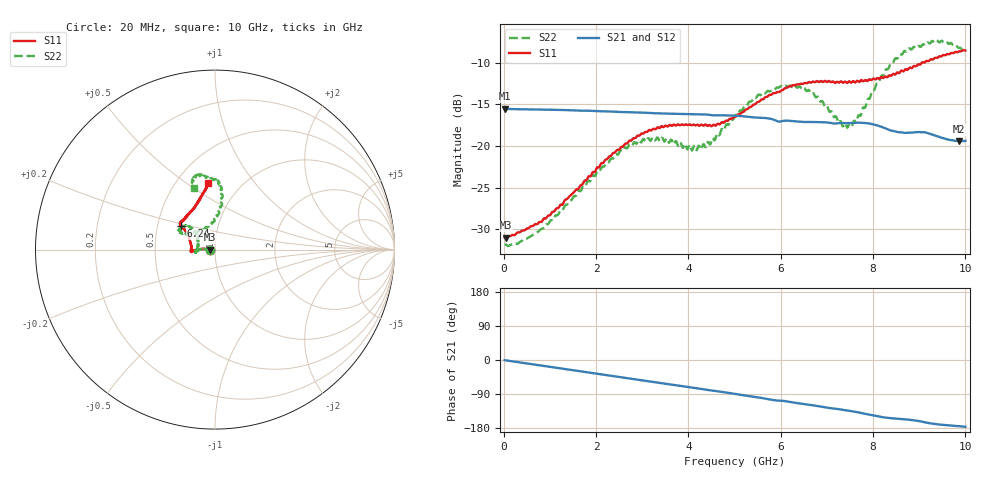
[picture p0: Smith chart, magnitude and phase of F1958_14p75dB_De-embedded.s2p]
! Integrated Device Technology
! Corporate Headquarters
! 6024 Silver Creek Valley Road
! San Jose, CA 95138  USA
! Phone:  1-408-284-8200
! Toll Free:  1-800-223-1366
! Webpage:  http://www.idt.com/
! Timing and RF Division
! 515 Groton Road, Suite 102
! Westford, MA 01886-6024
! Device:  F1958
! Description: 7-bit 0.25 dB Digital Step Attenuator
! Frequency:  0.001 -  6.000 GHz
! Package:  4x4 mm Thin QFN Plastic Package: 24 pin
! Ports:  2 RF, 12 DC
!  Pin  1  = D0
!  Pin  2  = VDD
!  Pin  3  = VMODE
!  Pin  4  = GND
!  Pin  5  = RF1  =  Port 1
!  Pin  6  = GND
!  Pin  7  = GND
!  Pin  8  = GND
!  Pin  9  = GND
!  Pin 10  = GND
!  Pin 11  = GND
!  Pin 12  = GND
!  Pin 13  = GND
!  Pin 14  = RF2  =  Port 2
!  Pin 15  = GND
!  Pin 16  = LE
!  Pin 17  = CLK
!  Pin 18  = DATA
!  Pin 19  = D6
!  Pin 20  = D5
!  Pin 21  = D4
!  Pin 22  = D3
!  Pin 23  = D2
!  Pin 24  = D1
! State:  59
! Atten State:  14.75 dB
! Voltage:  +3.30 Volts
! Current:  0.258 mA
! Data:  The device was measured on a F1958 evaluation board which has
!  individual transmission lines to the RF pins.  Data was collected
!  using a calibrated network analyzer.  The evaluation board was
!  de-embedded using Automatic Fixture Removal (AFR).
!  The reference plane is the edge of the package pin.
! Misc:
!  Action Tracker AT0419
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# GHz S dB R 50
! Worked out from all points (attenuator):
!   500 points, 20 MHz to 10 GHz, reference 50 ohm
!   highest |S21| = -15.54 dB at 20 MHz (marker M1); lowest = -19.4 dB at 9.86 GHz (marker M2)
!   lowest |S11| = -31.0 dB at 40 MHz (marker M3), VSWR 1.06, Z = 47.3 - j0.0733 ohm
!   |S11| at or under -10 dB: start of sweep to 9.059 GHz
!   |S22| runs from -32.0 to -7.3 dB; largest |S21 - S12| = 0.00054
!   S11 on the Smith chart (normalised r, x): 20 MHz: 0.95, -0.00; 6.24 GHz: 0.66, +0.18; 10 GHz: 0.70, +0.61
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0.02  -30.98 -178.4  -15.54 -0.5  -15.54 -0.4  -31.87 -178.5
0.04  -31.00 -178.4  -15.55 -0.9  -15.55 -0.8  -31.83 -177.8
0.32  -30.38 177.8  -15.59 -6.0  -15.59 -5.9  -31.69 177.8
0.84  -28.97 176.2  -15.64 -15.3  -15.63 -15.3  -29.94 178.2
1.7  -24.66 177.0  -15.77 -30.6  -15.76 -30.6  -25.03 177.2
2.62  -19.81 -179.4  -15.94 -47.0  -15.92 -47.0  -20.19 -177.3
2.92  -18.76 -176.9  -15.99 -52.3  -15.98 -52.4  -19.33 -174.9
3.36  -17.84 -174.7  -16.09 -60.1  -16.09 -60.3  -19.27 -170.9
4.24  -17.59 179.8  -16.21 -75.6  -16.23 -75.6  -20.01 166.8
4.5  -17.65 173.8  -16.31 -80.5  -16.32 -80.6  -19.40 151.6
5.02  -16.51 159.4  -16.37 -89.7  -16.38 -89.7  -16.28 138.3
5.54  -14.67 149.3  -16.61 -99.3  -16.62 -99.3  -13.87 139.6
6.24  -12.79 145.2  -17.01 -111.6  -17.02 -111.6  -12.91 150.9
6.68  -12.32 143.2  -17.13 -119.2  -17.15 -119.1  -13.70 152.7
7.3  -12.25 136.8  -17.26 -130.5  -17.26 -130.4  -17.01 131.3
7.5  -12.29 134.0  -17.27 -134.3  -17.27 -134.2  -17.33 113.2
7.68  -12.26 130.9  -17.20 -138.2  -17.20 -138.1  -16.35 96.6
8.34  -11.56 115.1  -18.05 -153.1  -18.05 -153.2  -10.64 81.8
8.68  -10.92 108.5  -18.43 -156.4  -18.42 -156.4  -8.58 86.4
9.26  -9.59 100.8  -18.62 -167.5  -18.61 -167.6  -7.52 99.2
9.86  -8.65 96.4  -19.43 -174.5  -19.46 -174.4  -8.23 108.3
10  -8.55 96.4  -19.39 -176.2  -19.42 -176.0  -8.76 109.1
